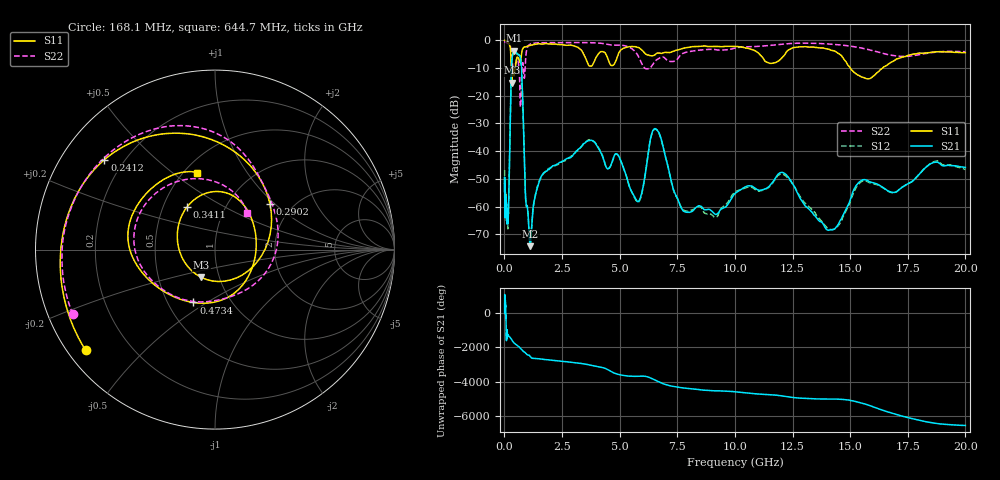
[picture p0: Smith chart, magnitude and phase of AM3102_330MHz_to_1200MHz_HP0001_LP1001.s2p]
! Date/Time: Tue, Sep 11, 2018 5:10 PM
! Network Analyzer: Agilent Technologies E8362B Rev: A.07.50.63
! Sweep from 0.010 to 20.000 GHz, 1601 Points, Sweep Type: LOG
! Power Supply: 4.949 V, 0.001 A
# Hz S DB R 50
!freq MagS11 AngS11 MagS21 AngS21 MagS12 AngS12 MagS22 AngS22
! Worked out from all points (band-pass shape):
!   1601 points, 10 MHz to 20 GHz, reference 50 ohm
!   highest |S21| = -3.72 dB at 434.6 MHz (marker M1); lowest = -74.3 dB at 1.119 GHz (marker M2)
!   |S21| within 3 dB of the highest: 329.4 MHz to 701.9 MHz (372.4 MHz wide, 72.2 % of centre)
!   lowest |S11| = -15.3 dB at 316.2 MHz (marker M3), VSWR 1.42, Z = 41.1 - j13.1 ohm
!   |S11| at or under -10 dB: 296 MHz to 350.9 MHz (54.87 MHz wide, 17 % of centre); 368.1 MHz to 472.4 MHz (104.4 MHz wide, 24.8 % of centre); 15.01 GHz to 16.4 GHz (1.394 GHz wide, 8.88 % of centre)
!   |S22| runs from -24.1 to -0.3 dB; largest |S21 - S12| = 0.012
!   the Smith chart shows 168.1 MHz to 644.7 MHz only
!   S11 on the Smith chart (normalised r, x): 168.1 MHz: 0.05, -0.34; 241.2 MHz: 0.13, +0.35; 290.2 MHz: 1.55, +0.93; 341.1 MHz: 0.66, +0.34; 473.4 MHz: 0.67, -0.44; 644.7 MHz: 0.58, +0.62
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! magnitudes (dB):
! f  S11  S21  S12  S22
! 10 MHz  0.0  -51.8  -46.9  -0.3
! 35.55 MHz  0.0  -63.0  -60.5  -0.5
! 126.4 MHz  -0.4  -63.0  -63.7  -1.0
! 168.1 MHz  -0.8  -62.2  -64.2  -1.2
! 241.2 MHz  -2.0  -35.3  -35.4  -1.8
! 290.2 MHz  -8.0  -14.6  -14.7  -3.6
! 316.2 MHz  -15.3  -8.2  -8.2  -6.1
! 341.1 MHz  -10.9  -5.9  -6.0  -8.0
! 434.6 MHz  -12.0  -3.7  -3.8  -10.4
! 447.2 MHz  -11.3  -3.7  -3.8  -9.9
! 473.4 MHz  -9.9  -3.9  -3.9  -8.8
! 644.7 MHz  -7.1  -5.3  -5.3  -11.3
! 702.3 MHz  -7.5  -6.7  -6.8  -24.1
! 1.119 GHz  -1.8  -74.3  -73.8  -1.3
! 1.59 GHz  -1.3  -49.2  -49.4  -0.8
! 3.757 GHz  -9.3  -36.0  -35.9  -0.8
! 5.652 GHz  -2.2  -56.6  -56.9  -3.9
! 6.549 GHz  -5.1  -31.9  -32.1  -7.4
! 7.958 GHz  -2.5  -62.1  -61.7  -4.1
! 12.03 GHz  -6.3  -47.7  -48.2  -1.4
! 14.14 GHz  -3.4  -68.4  -68.3  -1.3
! 20 GHz  -4.4  -45.9  -46.6  -4.1
